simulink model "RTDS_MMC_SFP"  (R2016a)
settings: Solver=FixedStepAuto  StartTime=0.0  StopTime=0.4  RelTol=1e-3
PreLoadFcn:
  | % --- DO NOT REMOVE THIS CODE (2024.3.b1) ---
  |     % create Simulink variants
  |     if not(exist('variant_simulation', 'var'))
  |         variant_simulation = Simulink.Variant('SIMULINK_MODE==0');
  |     end
  |     if not(exist('variant_generation', 'var'))
  |         variant_generation = Simulink.Variant('SIMULINK_MODE==1');
  |     end
  | 
  |     % check SDK version
  |     required_lib_version = 3900.3;
  |     required_lib_ver_str = '2024.3';
  |     lib_path = [getenv('IX_SIMULINK_ACG_BB_3') '\simulink\blocks\BoomBox.slx'];
  |     if exist(lib_path, 'file')
  |         lib_version = str2double(Simulink.MDLInfo(lib_path).ModelVersion); % fullpath to avoid getting shadowing files
  |         if lib_version < required_lib_version || isnan(lib_version)
  |             error(['The model ''' bdroot ''' has been saved with a more recent version of ACG SDK (' required_lib_ver_str ') and might not work as expected. <a href="matlab:private_end_string = ''--- PLACE YOUR CODE BELOW THIS LINE ---'';private_fcn = get_param(bdroot, ''PreLoadFcn'');private_end_index = strfind(private_fcn, private_end_string);set_param(bdroot, ''PreLoadFcn'', strtrim(private_fcn(private_end_index(end)+length(private_end_string):end)));private_fcn = get_param(bdroot, ''PostLoadFcn'');private_end_index = strfind(private_fcn, private_end_string);set_param(bdroot, ''PostLoadFcn'', strtrim(private_fcn(private_end_index(end)+length(private_end_string):end)));private_fcn = get_param(bdroot, ''InitFcn'');private_end_index = strfind(private_fcn, private_end_string);set_param(bdroot, ''InitFcn'', strtrim(private_fcn(private_end_index(end)+length(private_end_string):end)));clear private_end_string private_fcn private_end_index;open(bdroot);">Click here</a> to continue anyway, or download the latest version of the SDK at <a href="www.imperix.com/downloads">www.imperix.ch/downloads</a>.']);
  |         end
  |     elseif exist(getenv('IX_SIMULINK_ACG_BB_3'), 'dir')
  |         error(['Library file for imperix ACG SDK not found in path ''' lib_path '''. Please try to re-install ACG SDK (<a href="www.imperix.com/downloads">www.imperix.ch/downloads</a>).']);
  |     else
  |         error('ACG SDK is not installed on this computer and the model will not work as expected. Please download ACG SDK at <a href="www.imperix.com/downloads">www.imperix.ch/downloads</a>, install it, and reopen the model.');
  |     end
  |     clear required_lib_version required_lib_ver_str lib_path lib_version;
  | 
  |     ix_acg_path = getenv('IX_SIMULINK_ACG_BB_3');
  |     addpath(fullfile(ix_acg_path, 'simulink\target'));
  |     addpath(fullfile(ix_acg_path, 'simulink\blocks'));
  |     addpath(fullfile(ix_acg_path, 'simulink\functions'));
  |     sl_refresh_customizations;
  |     clear ix_acg_path;
  | 
  |     % The SIMULINK_MODE variable is created in the base
  |     % workspace in the PostLoadFcn from the block whose id is kb0101
  |     % All opened models share a common variant configuration.
  | 
  |     Model_PreLoadFcn(bdroot);
  | % --- PLACE YOUR CODE BELOW THIS LINE ---
PostLoadFcn:
  | % --- DO NOT REMOVE THIS CODE (2024.3.b1) ---
  |     % change the execution mode of simulink depending on the radio button:
  |     if(strcmp('Automated Code Generation',get_param(Find_imperix_blocks(bdroot,'Configuration'),'SLMODE')))
  |         assignin('base', 'SIMULINK_MODE', 1);
  |     else
  |         assignin('base', 'SIMULINK_MODE', 0);
  |     end
  | 
  |     Model_PostLoadFcn(bdroot);
  | % --- PLACE YOUR CODE BELOW THIS LINE ---
InitFcn:
  | % --- DO NOT REMOVE THIS CODE (2024.3.b1) ---
  |     % check SDK version
  |     required_lib_version = 3900.3;
  |     required_lib_ver_str = '2024.3';
  |     lib_path = [getenv('IX_SIMULINK_ACG_BB_3') '\simulink\blocks\BoomBox.slx'];
  |     if exist(lib_path, 'file')
  |         lib_version = str2double(Simulink.MDLInfo(lib_path).ModelVersion); % fullpath to avoid getting shadowing files
  |         if lib_version < required_lib_version || isnan(lib_version)
  |             error(['The model ''' bdroot ''' has been saved with a more recent version of ACG SDK (' required_lib_ver_str ') and might not work as expected. <a href="matlab:private_end_string = ''--- PLACE YOUR CODE BELOW THIS LINE ---'';private_fcn = get_param(bdroot, ''PreLoadFcn'');private_end_index = strfind(private_fcn, private_end_string);set_param(bdroot, ''PreLoadFcn'', strtrim(private_fcn(private_end_index(end)+length(private_end_string):end)));private_fcn = get_param(bdroot, ''PostLoadFcn'');private_end_index = strfind(private_fcn, private_end_string);set_param(bdroot, ''PostLoadFcn'', strtrim(private_fcn(private_end_index(end)+length(private_end_string):end)));private_fcn = get_param(bdroot, ''InitFcn'');private_end_index = strfind(private_fcn, private_end_string);set_param(bdroot, ''InitFcn'', strtrim(private_fcn(private_end_index(end)+length(private_end_string):end)));clear private_end_string private_fcn private_end_index;open(bdroot);">Click here</a> to continue anyway, or download the latest version of the SDK at <a href="www.imperix.com/downloads">www.imperix.ch/downloads</a>.']);
  |         end
  |     elseif exist(getenv('IX_SIMULINK_ACG_BB_3'), 'dir')
  |         error(['Library file for imperix ACG SDK not found in path ''' lib_path '''. Please try to re-install ACG SDK (<a href="www.imperix.com/downloads">www.imperix.ch/downloads</a>).']);
  |     else
  |         error('ACG SDK is not installed on this computer and the model will not work as expected. Please download ACG SDK at <a href="www.imperix.com/downloads">www.imperix.ch/downloads</a>, install it, and reopen the model.');
  |     end
  |     clear required_lib_version required_lib_ver_str lib_path lib_version;
  | 
  |     Model_InitFcn(bdroot);
  | % --- PLACE YOUR CODE BELOW THIS LINE ---
model workspace (MAT data in the model file):
  CTRLPERIOD = 0.0002
  TSAMPLE = 2e-06
  global_CLK_number = 0
  global_INT_number = 1
  global_SVM_instance_id = 0
  global_can_baud_rate = '1000000'
  global_comp_time = 0.2
  global_cycle_delay = 8e-05
  global_ip_addresses : cell (value not decoded)
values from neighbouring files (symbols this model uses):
  Ki_Vleg = 1/Ti    (= 2.95256991686)    [RTDS_MMC_SFP_init.m]
  Kp_Vleg = Tn/Ti    (= 0.14880952381)    [RTDS_MMC_SFP_init.m]
  N = 4    [RTDS_MMC_SFP_init.m]
  scale_factor = 0.5^16    (= 1.52587890625e-05)    [RTDS_MMC_SFP_init.m]
  Tsw = 1/fsw    (= 0.0008)    [RTDS_MMC_SFP_init.m]
  Vsm_max = 250    [RTDS_MMC_SFP_init.m]
undefined symbols (not defined in the file or in its folder): B, Board, Box, channel, DT, lane, Micro, ns, PRO, RCP, TPI, Vf
libraries: BoomBox x183, simulink x55
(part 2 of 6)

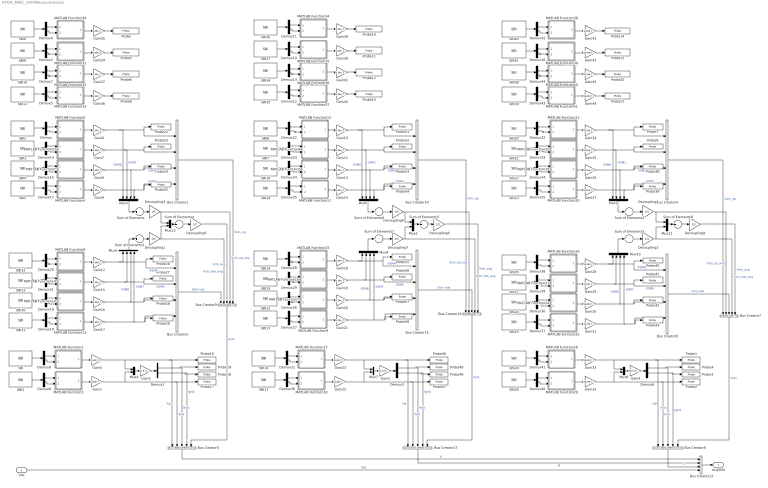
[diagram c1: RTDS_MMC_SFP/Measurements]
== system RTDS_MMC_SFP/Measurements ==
  Vdc : Inport
  Bus Creator{1..2,4,6,13..15} (7 alike) : BusCreator  Inputs=4
  Bus Creator{5,7..9,16..17} (6 alike) : BusCreator  Inputs=5
  Decoupling{1..4,7..8} (6 alike) : Gain  Gain=1/4
  Decoupling5 : Gain  Gain=1/2
  Decoupling6 : Gain  Gain=1/2
  Decoupling9 : Gain  Gain=1/2
  Demux{,1..44} (45 alike) : Demux  Outputs=2
  Gain{1,5..45} (42 alike) : Gain  Gain=scale_factor  OutDataTypeStr=single
  Gain2 : Gain  Gain=[0.5 0.5 ; 1 -1]  Multiplication=Matrix(K*u)
  Gain3 : Gain  Gain=[0.5 0.5 ; 1 -1]  Multiplication=Matrix(K*u)
  Gain4 : Gain  Gain=[0.5 0.5 ; 1 -1]  Multiplication=Matrix(K*u)
  MATLAB Function0 : MATLAB Function  TreatAsAtomicUnit=on
  MATLAB Function1 : MATLAB Function  TreatAsAtomicUnit=on
  MATLAB Function10 : MATLAB Function  TreatAsAtomicUnit=on
  MATLAB Function11 : MATLAB Function  TreatAsAtomicUnit=on
  MATLAB Function12 : MATLAB Function  TreatAsAtomicUnit=on
  MATLAB Function13 : MATLAB Function  TreatAsAtomicUnit=on
  MATLAB Function14 : MATLAB Function  TreatAsAtomicUnit=on
  MATLAB Function15 : MATLAB Function  TreatAsAtomicUnit=on
  MATLAB Function16 : MATLAB Function  TreatAsAtomicUnit=on
  MATLAB Function17 : MATLAB Function  TreatAsAtomicUnit=on
  MATLAB Function18 : MATLAB Function  TreatAsAtomicUnit=on
  MATLAB Function19 : MATLAB Function  TreatAsAtomicUnit=on
  MATLAB Function2 : MATLAB Function  TreatAsAtomicUnit=on
  MATLAB Function20 : MATLAB Function  TreatAsAtomicUnit=on
  MATLAB Function21 : MATLAB Function  TreatAsAtomicUnit=on
  MATLAB Function22 : MATLAB Function  TreatAsAtomicUnit=on
  MATLAB Function23 : MATLAB Function  TreatAsAtomicUnit=on
  MATLAB Function24 : MATLAB Function  TreatAsAtomicUnit=on
  MATLAB Function25 : MATLAB Function  TreatAsAtomicUnit=on
  MATLAB Function26 : MATLAB Function  TreatAsAtomicUnit=on
  MATLAB Function27 : MATLAB Function  TreatAsAtomicUnit=on
  MATLAB Function28 : MATLAB Function  TreatAsAtomicUnit=on
  MATLAB Function29 : MATLAB Function  TreatAsAtomicUnit=on
  MATLAB Function3 : MATLAB Function  TreatAsAtomicUnit=on
  MATLAB Function30 : MATLAB Function  TreatAsAtomicUnit=on
  MATLAB Function31 : MATLAB Function  TreatAsAtomicUnit=on
  MATLAB Function32 : MATLAB Function  TreatAsAtomicUnit=on
  MATLAB Function33 : MATLAB Function  TreatAsAtomicUnit=on
  MATLAB Function34 : MATLAB Function  TreatAsAtomicUnit=on
  MATLAB Function35 : MATLAB Function  TreatAsAtomicUnit=on
  MATLAB Function36 : MATLAB Function  TreatAsAtomicUnit=on
  MATLAB Function37 : MATLAB Function  TreatAsAtomicUnit=on
  MATLAB Function38 : MATLAB Function  TreatAsAtomicUnit=on
  MATLAB Function39 : MATLAB Function  TreatAsAtomicUnit=on
  MATLAB Function4 : MATLAB Function  TreatAsAtomicUnit=on
  MATLAB Function40 : MATLAB Function  TreatAsAtomicUnit=on
  MATLAB Function41 : MATLAB Function  TreatAsAtomicUnit=on
  MATLAB Function5 : MATLAB Function  TreatAsAtomicUnit=on
  MATLAB Function6 : MATLAB Function  TreatAsAtomicUnit=on
  MATLAB Function7 : MATLAB Function  TreatAsAtomicUnit=on
  MATLAB Function8 : MATLAB Function  TreatAsAtomicUnit=on
  MATLAB Function9 : MATLAB Function  TreatAsAtomicUnit=on
  Mux{1,3,5..6,9..10} (6 alike) : Mux
  Mux{2,4,7..8,11..12} (6 alike) : Mux  Inputs=2
  Probe : BoomBox/Probe  VARNAME=v_leg_1  EVALUATE=Literal  DATATYPE=single  CAN_ENABLED=off  CAN_ADDRESS=0  CAN_TX_FREQ=10  init_baudrate=0  CAN_BAUDRATE=1000000  can_endianness=Little-endian  ETH_ENABLED=off  ETH_PORT=2000  ETH_IP_LIST=IP address 0  eth_endianness=Little-endian  ETH_TX_FREQ=10  init_ip=0  KBID=kb0502  CAN_BIG_ENDIAN=0  ETH_BIG_ENDIAN=0  ETH_IP_SFCN=empty  CAN_MB_ID=0  ETH_MB_ID=1  RESIZE=0
  Probe1 : BoomBox/Probe  VARNAME=Iup_C  EVALUATE=Literal  DATATYPE=single  CAN_ENABLED=off  CAN_ADDRESS=0  CAN_TX_FREQ=10  init_baudrate=0  CAN_BAUDRATE=1000000  can_endianness=Little-endian  ETH_ENABLED=off  ETH_PORT=2000  ETH_IP_LIST=IP address 0  eth_endianness=Little-endian  ETH_TX_FREQ=10  init_ip=0  KBID=kb0502  CAN_BIG_ENDIAN=0  ETH_BIG_ENDIAN=0  ETH_IP_SFCN=empty  CAN_MB_ID=0  ETH_MB_ID=0  RESIZE=0
  Probe10 : BoomBox/Probe  VARNAME=v_leg_3  EVALUATE=Literal  DATATYPE=single  CAN_ENABLED=off  CAN_ADDRESS=0  CAN_TX_FREQ=10  init_baudrate=0  CAN_BAUDRATE=1000000  can_endianness=Little-endian  ETH_ENABLED=off  ETH_PORT=2000  ETH_IP_LIST=IP address 0  eth_endianness=Little-endian  ETH_TX_FREQ=10  init_ip=0  KBID=kb0502  CAN_BIG_ENDIAN=0  ETH_BIG_ENDIAN=0  ETH_IP_SFCN=empty  CAN_MB_ID=0  ETH_MB_ID=1  RESIZE=0
  Probe11 : BoomBox/Probe  VARNAME=v_valves_3  EVALUATE=Literal  DATATYPE=single  CAN_ENABLED=off  CAN_ADDRESS=0  CAN_TX_FREQ=10  init_baudrate=0  CAN_BAUDRATE=1000000  can_endianness=Little-endian  ETH_ENABLED=off  ETH_PORT=2000  ETH_IP_LIST=IP address 0  eth_endianness=Little-endian  ETH_TX_FREQ=10  init_ip=0  KBID=kb0502  CAN_BIG_ENDIAN=0  ETH_BIG_ENDIAN=0  ETH_IP_SFCN=empty  CAN_MB_ID=0  ETH_MB_ID=1  RESIZE=0
  Probe12 : BoomBox/Probe  VARNAME=v_leg_4  EVALUATE=Literal  DATATYPE=single  CAN_ENABLED=off  CAN_ADDRESS=0  CAN_TX_FREQ=10  init_baudrate=0  CAN_BAUDRATE=1000000  can_endianness=Little-endian  ETH_ENABLED=off  ETH_PORT=2000  ETH_IP_LIST=IP address 0  eth_endianness=Little-endian  ETH_TX_FREQ=10  init_ip=0  KBID=kb0502  CAN_BIG_ENDIAN=0  ETH_BIG_ENDIAN=0  ETH_IP_SFCN=empty  CAN_MB_ID=0  ETH_MB_ID=1  RESIZE=0
  Probe13 : BoomBox/Probe  VARNAME=v_valves_4  EVALUATE=Literal  DATATYPE=single  CAN_ENABLED=off  CAN_ADDRESS=0  CAN_TX_FREQ=10  init_baudrate=0  CAN_BAUDRATE=1000000  can_endianness=Little-endian  ETH_ENABLED=off  ETH_PORT=2000  ETH_IP_LIST=IP address 0  eth_endianness=Little-endian  ETH_TX_FREQ=10  init_ip=0  KBID=kb0502  CAN_BIG_ENDIAN=0  ETH_BIG_ENDIAN=0  ETH_IP_SFCN=empty  CAN_MB_ID=0  ETH_MB_ID=1  RESIZE=0
  Probe14 : BoomBox/Probe  VARNAME=v_leg_5  EVALUATE=Literal  DATATYPE=single  CAN_ENABLED=off  CAN_ADDRESS=0  CAN_TX_FREQ=10  init_baudrate=0  CAN_BAUDRATE=1000000  can_endianness=Little-endian  ETH_ENABLED=off  ETH_PORT=2000  ETH_IP_LIST=IP address 0  eth_endianness=Little-endian  ETH_TX_FREQ=10  init_ip=0  KBID=kb0502  CAN_BIG_ENDIAN=0  ETH_BIG_ENDIAN=0  ETH_IP_SFCN=empty  CAN_MB_ID=0  ETH_MB_ID=1  RESIZE=0
  Probe15 : BoomBox/Probe  VARNAME=v_valves_5  EVALUATE=Literal  DATATYPE=single  CAN_ENABLED=off  CAN_ADDRESS=0  CAN_TX_FREQ=10  init_baudrate=0  CAN_BAUDRATE=1000000  can_endianness=Little-endian  ETH_ENABLED=off  ETH_PORT=2000  ETH_IP_LIST=IP address 0  eth_endianness=Little-endian  ETH_TX_FREQ=10  init_ip=0  KBID=kb0502  CAN_BIG_ENDIAN=0  ETH_BIG_ENDIAN=0  ETH_IP_SFCN=empty  CAN_MB_ID=0  ETH_MB_ID=1  RESIZE=0
  Probe16 : BoomBox/Probe  VARNAME=Iup_A  EVALUATE=Literal  DATATYPE=single  CAN_ENABLED=off  CAN_ADDRESS=0  CAN_TX_FREQ=10  init_baudrate=0  CAN_BAUDRATE=1000000  can_endianness=Little-endian  ETH_ENABLED=off  ETH_PORT=2000  ETH_IP_LIST=IP address 0  eth_endianness=Little-endian  ETH_TX_FREQ=10  init_ip=0  KBID=kb0502  CAN_BIG_ENDIAN=0  ETH_BIG_ENDIAN=0  ETH_IP_SFCN=empty  CAN_MB_ID=0  ETH_MB_ID=0  RESIZE=0
  Probe17 : BoomBox/Probe  VARNAME=Ilow_A  EVALUATE=Literal  DATATYPE=single  CAN_ENABLED=off  CAN_ADDRESS=0  CAN_TX_FREQ=10  init_baudrate=0  CAN_BAUDRATE=1000000  can_endianness=Little-endian  ETH_ENABLED=off  ETH_PORT=2000  ETH_IP_LIST=IP address 0  eth_endianness=Little-endian  ETH_TX_FREQ=10  init_ip=0  KBID=kb0502  CAN_BIG_ENDIAN=0  ETH_BIG_ENDIAN=0  ETH_IP_SFCN=empty  CAN_MB_ID=0  ETH_MB_ID=0  RESIZE=0
  Probe18 : BoomBox/Probe  VARNAME=Ig_A  EVALUATE=Literal  DATATYPE=single  CAN_ENABLED=off  CAN_ADDRESS=0  CAN_TX_FREQ=10  init_baudrate=0  CAN_BAUDRATE=1000000  can_endianness=Little-endian  ETH_ENABLED=off  ETH_PORT=2000  ETH_IP_LIST=IP address 0  eth_endianness=Little-endian  ETH_TX_FREQ=10  init_ip=0  KBID=kb0502  CAN_BIG_ENDIAN=0  ETH_BIG_ENDIAN=0  ETH_IP_SFCN=empty  CAN_MB_ID=0  ETH_MB_ID=0  RESIZE=0
  Probe19 : BoomBox/Probe  VARNAME=Ibus_A  EVALUATE=Literal  DATATYPE=single  CAN_ENABLED=off  CAN_ADDRESS=0  CAN_TX_FREQ=10  init_baudrate=0  CAN_BAUDRATE=1000000  can_endianness=Little-endian  ETH_ENABLED=off  ETH_PORT=2000  ETH_IP_LIST=IP address 0  eth_endianness=Little-endian  ETH_TX_FREQ=10  init_ip=0  KBID=kb0502  CAN_BIG_ENDIAN=0  ETH_BIG_ENDIAN=0  ETH_IP_SFCN=empty  CAN_MB_ID=0  ETH_MB_ID=0  RESIZE=0
  Probe2 : BoomBox/Probe  VARNAME=Ilow_C  EVALUATE=Literal  DATATYPE=single  CAN_ENABLED=off  CAN_ADDRESS=0  CAN_TX_FREQ=10  init_baudrate=0  CAN_BAUDRATE=1000000  can_endianness=Little-endian  ETH_ENABLED=off  ETH_PORT=2000  ETH_IP_LIST=IP address 0  eth_endianness=Little-endian  ETH_TX_FREQ=10  init_ip=0  KBID=kb0502  CAN_BIG_ENDIAN=0  ETH_BIG_ENDIAN=0  ETH_IP_SFCN=empty  CAN_MB_ID=0  ETH_MB_ID=0  RESIZE=0
  Probe20 : BoomBox/Probe  VARNAME=v_leg_6  EVALUATE=Literal  DATATYPE=single  CAN_ENABLED=off  CAN_ADDRESS=0  CAN_TX_FREQ=10  init_baudrate=0  CAN_BAUDRATE=1000000  can_endianness=Little-endian  ETH_ENABLED=off  ETH_PORT=2000  ETH_IP_LIST=IP address 0  eth_endianness=Little-endian  ETH_TX_FREQ=10  init_ip=0  KBID=kb0502  CAN_BIG_ENDIAN=0  ETH_BIG_ENDIAN=0  ETH_IP_SFCN=empty  CAN_MB_ID=0  ETH_MB_ID=1  RESIZE=0
  Probe21 : BoomBox/Probe  VARNAME=v_valves_6  EVALUATE=Literal  DATATYPE=single  CAN_ENABLED=off  CAN_ADDRESS=0  CAN_TX_FREQ=10  init_baudrate=0  CAN_BAUDRATE=1000000  can_endianness=Little-endian  ETH_ENABLED=off  ETH_PORT=2000  ETH_IP_LIST=IP address 0  eth_endianness=Little-endian  ETH_TX_FREQ=10  init_ip=0  KBID=kb0502  CAN_BIG_ENDIAN=0  ETH_BIG_ENDIAN=0  ETH_IP_SFCN=empty  CAN_MB_ID=0  ETH_MB_ID=1  RESIZE=0
  Probe22 : BoomBox/Probe  VARNAME=Vsm_A0  EVALUATE=Literal  DATATYPE=single  CAN_ENABLED=off  CAN_ADDRESS=0  CAN_TX_FREQ=10  init_baudrate=0  CAN_BAUDRATE=1000000  can_endianness=Little-endian  ETH_ENABLED=off  ETH_PORT=2000  ETH_IP_LIST=IP address 0  eth_endianness=Little-endian  ETH_TX_FREQ=10  init_ip=0  KBID=kb0502  CAN_BIG_ENDIAN=0  ETH_BIG_ENDIAN=0  ETH_IP_SFCN=empty  CAN_MB_ID=0  ETH_MB_ID=0  RESIZE=0
  Probe23 : BoomBox/Probe  VARNAME=Vsm_A1  EVALUATE=Literal  DATATYPE=single  CAN_ENABLED=off  CAN_ADDRESS=0  CAN_TX_FREQ=10  init_baudrate=0  CAN_BAUDRATE=1000000  can_endianness=Little-endian  ETH_ENABLED=off  ETH_PORT=2000  ETH_IP_LIST=IP address 0  eth_endianness=Little-endian  ETH_TX_FREQ=10  init_ip=0  KBID=kb0502  CAN_BIG_ENDIAN=0  ETH_BIG_ENDIAN=0  ETH_IP_SFCN=empty  CAN_MB_ID=0  ETH_MB_ID=0  RESIZE=0
  Probe24 : BoomBox/Probe  VARNAME=Vsm_A2  EVALUATE=Literal  DATATYPE=single  CAN_ENABLED=off  CAN_ADDRESS=0  CAN_TX_FREQ=10  init_baudrate=0  CAN_BAUDRATE=1000000  can_endianness=Little-endian  ETH_ENABLED=off  ETH_PORT=2000  ETH_IP_LIST=IP address 0  eth_endianness=Little-endian  ETH_TX_FREQ=10  init_ip=0  KBID=kb0502  CAN_BIG_ENDIAN=0  ETH_BIG_ENDIAN=0  ETH_IP_SFCN=empty  CAN_MB_ID=0  ETH_MB_ID=0  RESIZE=0
  Probe25 : BoomBox/Probe  VARNAME=Vsm_A3  EVALUATE=Literal  DATATYPE=single  CAN_ENABLED=off  CAN_ADDRESS=0  CAN_TX_FREQ=10  init_baudrate=0  CAN_BAUDRATE=1000000  can_endianness=Little-endian  ETH_ENABLED=off  ETH_PORT=2000  ETH_IP_LIST=IP address 0  eth_endianness=Little-endian  ETH_TX_FREQ=10  init_ip=0  KBID=kb0502  CAN_BIG_ENDIAN=0  ETH_BIG_ENDIAN=0  ETH_IP_SFCN=empty  CAN_MB_ID=0  ETH_MB_ID=0  RESIZE=0
  Probe26 : BoomBox/Probe  VARNAME=Vsm_A4  EVALUATE=Literal  DATATYPE=single  CAN_ENABLED=off  CAN_ADDRESS=0  CAN_TX_FREQ=10  init_baudrate=0  CAN_BAUDRATE=1000000  can_endianness=Little-endian  ETH_ENABLED=off  ETH_PORT=2000  ETH_IP_LIST=IP address 0  eth_endianness=Little-endian  ETH_TX_FREQ=10  init_ip=0  KBID=kb0502  CAN_BIG_ENDIAN=0  ETH_BIG_ENDIAN=0  ETH_IP_SFCN=empty  CAN_MB_ID=0  ETH_MB_ID=0  RESIZE=0
  Probe27 : BoomBox/Probe  VARNAME=Vsm_A5  EVALUATE=Literal  DATATYPE=single  CAN_ENABLED=off  CAN_ADDRESS=0  CAN_TX_FREQ=10  init_baudrate=0  CAN_BAUDRATE=1000000  can_endianness=Little-endian  ETH_ENABLED=off  ETH_PORT=2000  ETH_IP_LIST=IP address 0  eth_endianness=Little-endian  ETH_TX_FREQ=10  init_ip=0  KBID=kb0502  CAN_BIG_ENDIAN=0  ETH_BIG_ENDIAN=0  ETH_IP_SFCN=empty  CAN_MB_ID=0  ETH_MB_ID=0  RESIZE=0
  Probe28 : BoomBox/Probe  VARNAME=Vsm_A6  EVALUATE=Literal  DATATYPE=single  CAN_ENABLED=off  CAN_ADDRESS=0  CAN_TX_FREQ=10  init_baudrate=0  CAN_BAUDRATE=1000000  can_endianness=Little-endian  ETH_ENABLED=off  ETH_PORT=2000  ETH_IP_LIST=IP address 0  eth_endianness=Little-endian  ETH_TX_FREQ=10  init_ip=0  KBID=kb0502  CAN_BIG_ENDIAN=0  ETH_BIG_ENDIAN=0  ETH_IP_SFCN=empty  CAN_MB_ID=0  ETH_MB_ID=0  RESIZE=0
  Probe29 : BoomBox/Probe  VARNAME=Vsm_A7  EVALUATE=Literal  DATATYPE=single  CAN_ENABLED=off  CAN_ADDRESS=0  CAN_TX_FREQ=10  init_baudrate=0  CAN_BAUDRATE=1000000  can_endianness=Little-endian  ETH_ENABLED=off  ETH_PORT=2000  ETH_IP_LIST=IP address 0  eth_endianness=Little-endian  ETH_TX_FREQ=10  init_ip=0  KBID=kb0502  CAN_BIG_ENDIAN=0  ETH_BIG_ENDIAN=0  ETH_IP_SFCN=empty  CAN_MB_ID=0  ETH_MB_ID=0  RESIZE=0
  Probe3 : BoomBox/Probe  VARNAME=Ig_C  EVALUATE=Literal  DATATYPE=single  CAN_ENABLED=off  CAN_ADDRESS=0  CAN_TX_FREQ=10  init_baudrate=0  CAN_BAUDRATE=1000000  can_endianness=Little-endian  ETH_ENABLED=off  ETH_PORT=2000  ETH_IP_LIST=IP address 0  eth_endianness=Little-endian  ETH_TX_FREQ=10  init_ip=0  KBID=kb0502  CAN_BIG_ENDIAN=0  ETH_BIG_ENDIAN=0  ETH_IP_SFCN=empty  CAN_MB_ID=0  ETH_MB_ID=0  RESIZE=0
  Probe38 : BoomBox/Probe  VARNAME=Vsm_C2  EVALUATE=Literal  DATATYPE=single  CAN_ENABLED=off  CAN_ADDRESS=0  CAN_TX_FREQ=10  init_baudrate=0  CAN_BAUDRATE=1000000  can_endianness=Little-endian  ETH_ENABLED=off  ETH_PORT=2000  ETH_IP_LIST=IP address 0  eth_endianness=Little-endian  ETH_TX_FREQ=10  init_ip=0  KBID=kb0502  CAN_BIG_ENDIAN=0  ETH_BIG_ENDIAN=0  ETH_IP_SFCN=empty  CAN_MB_ID=0  ETH_MB_ID=0  RESIZE=0
  Probe39 : BoomBox/Probe  VARNAME=Vsm_C3  EVALUATE=Literal  DATATYPE=single  CAN_ENABLED=off  CAN_ADDRESS=0  CAN_TX_FREQ=10  init_baudrate=0  CAN_BAUDRATE=1000000  can_endianness=Little-endian  ETH_ENABLED=off  ETH_PORT=2000  ETH_IP_LIST=IP address 0  eth_endianness=Little-endian  ETH_TX_FREQ=10  init_ip=0  KBID=kb0502  CAN_BIG_ENDIAN=0  ETH_BIG_ENDIAN=0  ETH_IP_SFCN=empty  CAN_MB_ID=0  ETH_MB_ID=0  RESIZE=0
  Probe4 : BoomBox/Probe  VARNAME=Ibus_C  EVALUATE=Literal  DATATYPE=single  CAN_ENABLED=off  CAN_ADDRESS=0  CAN_TX_FREQ=10  init_baudrate=0  CAN_BAUDRATE=1000000  can_endianness=Little-endian  ETH_ENABLED=off  ETH_PORT=2000  ETH_IP_LIST=IP address 0  eth_endianness=Little-endian  ETH_TX_FREQ=10  init_ip=0  KBID=kb0502  CAN_BIG_ENDIAN=0  ETH_BIG_ENDIAN=0  ETH_IP_SFCN=empty  CAN_MB_ID=0  ETH_MB_ID=0  RESIZE=0
  Probe40 : BoomBox/Probe  VARNAME=Vsm_C4  EVALUATE=Literal  DATATYPE=single  CAN_ENABLED=off  CAN_ADDRESS=0  CAN_TX_FREQ=10  init_baudrate=0  CAN_BAUDRATE=1000000  can_endianness=Little-endian  ETH_ENABLED=off  ETH_PORT=2000  ETH_IP_LIST=IP address 0  eth_endianness=Little-endian  ETH_TX_FREQ=10  init_ip=0  KBID=kb0502  CAN_BIG_ENDIAN=0  ETH_BIG_ENDIAN=0  ETH_IP_SFCN=empty  CAN_MB_ID=0  ETH_MB_ID=0  RESIZE=0
  Probe41 : BoomBox/Probe  VARNAME=Vsm_C5  EVALUATE=Literal  DATATYPE=single  CAN_ENABLED=off  CAN_ADDRESS=0  CAN_TX_FREQ=10  init_baudrate=0  CAN_BAUDRATE=1000000  can_endianness=Little-endian  ETH_ENABLED=off  ETH_PORT=2000  ETH_IP_LIST=IP address 0  eth_endianness=Little-endian  ETH_TX_FREQ=10  init_ip=0  KBID=kb0502  CAN_BIG_ENDIAN=0  ETH_BIG_ENDIAN=0  ETH_IP_SFCN=empty  CAN_MB_ID=0  ETH_MB_ID=0  RESIZE=0
  Probe42 : BoomBox/Probe  VARNAME=Vsm_C6  EVALUATE=Literal  DATATYPE=single  CAN_ENABLED=off  CAN_ADDRESS=0  CAN_TX_FREQ=10  init_baudrate=0  CAN_BAUDRATE=1000000  can_endianness=Little-endian  ETH_ENABLED=off  ETH_PORT=2000  ETH_IP_LIST=IP address 0  eth_endianness=Little-endian  ETH_TX_FREQ=10  init_ip=0  KBID=kb0502  CAN_BIG_ENDIAN=0  ETH_BIG_ENDIAN=0  ETH_IP_SFCN=empty  CAN_MB_ID=0  ETH_MB_ID=0  RESIZE=0
  Probe43 : BoomBox/Probe  VARNAME=Vsm_C7  EVALUATE=Literal  DATATYPE=single  CAN_ENABLED=off  CAN_ADDRESS=0  CAN_TX_FREQ=10  init_baudrate=0  CAN_BAUDRATE=1000000  can_endianness=Little-endian  ETH_ENABLED=off  ETH_PORT=2000  ETH_IP_LIST=IP address 0  eth_endianness=Little-endian  ETH_TX_FREQ=10  init_ip=0  KBID=kb0502  CAN_BIG_ENDIAN=0  ETH_BIG_ENDIAN=0  ETH_IP_SFCN=empty  CAN_MB_ID=0  ETH_MB_ID=0  RESIZE=0
  Probe46 : BoomBox/Probe  VARNAME=Iup_B  EVALUATE=Literal  DATATYPE=single  CAN_ENABLED=off  CAN_ADDRESS=0  CAN_TX_FREQ=10  init_baudrate=0  CAN_BAUDRATE=1000000  can_endianness=Little-endian  ETH_ENABLED=off  ETH_PORT=2000  ETH_IP_LIST=IP address 0  eth_endianness=Little-endian  ETH_TX_FREQ=10  init_ip=0  KBID=kb0502  CAN_BIG_ENDIAN=0  ETH_BIG_ENDIAN=0  ETH_IP_SFCN=empty  CAN_MB_ID=0  ETH_MB_ID=0  RESIZE=0
  Probe47 : BoomBox/Probe  VARNAME=Ilow_B  EVALUATE=Literal  DATATYPE=single  CAN_ENABLED=off  CAN_ADDRESS=0  CAN_TX_FREQ=10  init_baudrate=0  CAN_BAUDRATE=1000000  can_endianness=Little-endian  ETH_ENABLED=off  ETH_PORT=2000  ETH_IP_LIST=IP address 0  eth_endianness=Little-endian  ETH_TX_FREQ=10  init_ip=0  KBID=kb0502  CAN_BIG_ENDIAN=0  ETH_BIG_ENDIAN=0  ETH_IP_SFCN=empty  CAN_MB_ID=0  ETH_MB_ID=0  RESIZE=0
  Probe48 : BoomBox/Probe  VARNAME=Ig_B  EVALUATE=Literal  DATATYPE=single  CAN_ENABLED=off  CAN_ADDRESS=0  CAN_TX_FREQ=10  init_baudrate=0  CAN_BAUDRATE=1000000  can_endianness=Little-endian  ETH_ENABLED=off  ETH_PORT=2000  ETH_IP_LIST=IP address 0  eth_endianness=Little-endian  ETH_TX_FREQ=10  init_ip=0  KBID=kb0502  CAN_BIG_ENDIAN=0  ETH_BIG_ENDIAN=0  ETH_IP_SFCN=empty  CAN_MB_ID=0  ETH_MB_ID=0  RESIZE=0
  Probe49 : BoomBox/Probe  VARNAME=Ibus_B  EVALUATE=Literal  DATATYPE=single  CAN_ENABLED=off  CAN_ADDRESS=0  CAN_TX_FREQ=10  init_baudrate=0  CAN_BAUDRATE=1000000  can_endianness=Little-endian  ETH_ENABLED=off  ETH_PORT=2000  ETH_IP_LIST=IP address 0  eth_endianness=Little-endian  ETH_TX_FREQ=10  init_ip=0  KBID=kb0502  CAN_BIG_ENDIAN=0  ETH_BIG_ENDIAN=0  ETH_IP_SFCN=empty  CAN_MB_ID=0  ETH_MB_ID=0  RESIZE=0
  Probe5 : BoomBox/Probe  VARNAME=v_valves_1  EVALUATE=Literal  DATATYPE=single  CAN_ENABLED=off  CAN_ADDRESS=0  CAN_TX_FREQ=10  init_baudrate=0  CAN_BAUDRATE=1000000  can_endianness=Little-endian  ETH_ENABLED=off  ETH_PORT=2000  ETH_IP_LIST=IP address 0  eth_endianness=Little-endian  ETH_TX_FREQ=10  init_ip=0  KBID=kb0502  CAN_BIG_ENDIAN=0  ETH_BIG_ENDIAN=0  ETH_IP_SFCN=empty  CAN_MB_ID=0  ETH_MB_ID=1  RESIZE=0
  Probe51 : BoomBox/Probe  VARNAME=Vsm_B0  EVALUATE=Literal  DATATYPE=single  CAN_ENABLED=off  CAN_ADDRESS=0  CAN_TX_FREQ=10  init_baudrate=0  CAN_BAUDRATE=1000000  can_endianness=Little-endian  ETH_ENABLED=off  ETH_PORT=2000  ETH_IP_LIST=IP address 0  eth_endianness=Little-endian  ETH_TX_FREQ=10  init_ip=0  KBID=kb0502  CAN_BIG_ENDIAN=0  ETH_BIG_ENDIAN=0  ETH_IP_SFCN=empty  CAN_MB_ID=0  ETH_MB_ID=0  RESIZE=0
  Probe52 : BoomBox/Probe  VARNAME=Vsm_B1  EVALUATE=Literal  DATATYPE=single  CAN_ENABLED=off  CAN_ADDRESS=0  CAN_TX_FREQ=10  init_baudrate=0  CAN_BAUDRATE=1000000  can_endianness=Little-endian  ETH_ENABLED=off  ETH_PORT=2000  ETH_IP_LIST=IP address 0  eth_endianness=Little-endian  ETH_TX_FREQ=10  init_ip=0  KBID=kb0502  CAN_BIG_ENDIAN=0  ETH_BIG_ENDIAN=0  ETH_IP_SFCN=empty  CAN_MB_ID=0  ETH_MB_ID=0  RESIZE=0
  Probe53 : BoomBox/Probe  VARNAME=Vsm_B2  EVALUATE=Literal  DATATYPE=single  CAN_ENABLED=off  CAN_ADDRESS=0  CAN_TX_FREQ=10  init_baudrate=0  CAN_BAUDRATE=1000000  can_endianness=Little-endian  ETH_ENABLED=off  ETH_PORT=2000  ETH_IP_LIST=IP address 0  eth_endianness=Little-endian  ETH_TX_FREQ=10  init_ip=0  KBID=kb0502  CAN_BIG_ENDIAN=0  ETH_BIG_ENDIAN=0  ETH_IP_SFCN=empty  CAN_MB_ID=0  ETH_MB_ID=0  RESIZE=0
  Probe54 : BoomBox/Probe  VARNAME=Vsm_B3  EVALUATE=Literal  DATATYPE=single  CAN_ENABLED=off  CAN_ADDRESS=0  CAN_TX_FREQ=10  init_baudrate=0  CAN_BAUDRATE=1000000  can_endianness=Little-endian  ETH_ENABLED=off  ETH_PORT=2000  ETH_IP_LIST=IP address 0  eth_endianness=Little-endian  ETH_TX_FREQ=10  init_ip=0  KBID=kb0502  CAN_BIG_ENDIAN=0  ETH_BIG_ENDIAN=0  ETH_IP_SFCN=empty  CAN_MB_ID=0  ETH_MB_ID=0  RESIZE=0
  Probe55 : BoomBox/Probe  VARNAME=Vsm_B4  EVALUATE=Literal  DATATYPE=single  CAN_ENABLED=off  CAN_ADDRESS=0  CAN_TX_FREQ=10  init_baudrate=0  CAN_BAUDRATE=1000000  can_endianness=Little-endian  ETH_ENABLED=off  ETH_PORT=2000  ETH_IP_LIST=IP address 0  eth_endianness=Little-endian  ETH_TX_FREQ=10  init_ip=0  KBID=kb0502  CAN_BIG_ENDIAN=0  ETH_BIG_ENDIAN=0  ETH_IP_SFCN=empty  CAN_MB_ID=0  ETH_MB_ID=0  RESIZE=0
  Probe56 : BoomBox/Probe  VARNAME=Vsm_B5  EVALUATE=Literal  DATATYPE=single  CAN_ENABLED=off  CAN_ADDRESS=0  CAN_TX_FREQ=10  init_baudrate=0  CAN_BAUDRATE=1000000  can_endianness=Little-endian  ETH_ENABLED=off  ETH_PORT=2000  ETH_IP_LIST=IP address 0  eth_endianness=Little-endian  ETH_TX_FREQ=10  init_ip=0  KBID=kb0502  CAN_BIG_ENDIAN=0  ETH_BIG_ENDIAN=0  ETH_IP_SFCN=empty  CAN_MB_ID=0  ETH_MB_ID=0  RESIZE=0
  Probe57 : BoomBox/Probe  VARNAME=Vsm_B6  EVALUATE=Literal  DATATYPE=single  CAN_ENABLED=off  CAN_ADDRESS=0  CAN_TX_FREQ=10  init_baudrate=0  CAN_BAUDRATE=1000000  can_endianness=Little-endian  ETH_ENABLED=off  ETH_PORT=2000  ETH_IP_LIST=IP address 0  eth_endianness=Little-endian  ETH_TX_FREQ=10  init_ip=0  KBID=kb0502  CAN_BIG_ENDIAN=0  ETH_BIG_ENDIAN=0  ETH_IP_SFCN=empty  CAN_MB_ID=0  ETH_MB_ID=0  RESIZE=0
  Probe58 : BoomBox/Probe  VARNAME=Vsm_B7  EVALUATE=Literal  DATATYPE=single  CAN_ENABLED=off  CAN_ADDRESS=0  CAN_TX_FREQ=10  init_baudrate=0  CAN_BAUDRATE=1000000  can_endianness=Little-endian  ETH_ENABLED=off  ETH_PORT=2000  ETH_IP_LIST=IP address 0  eth_endianness=Little-endian  ETH_TX_FREQ=10  init_ip=0  KBID=kb0502  CAN_BIG_ENDIAN=0  ETH_BIG_ENDIAN=0  ETH_IP_SFCN=empty  CAN_MB_ID=0  ETH_MB_ID=0  RESIZE=0
  Probe6 : BoomBox/Probe  VARNAME=v_leg_2  EVALUATE=Literal  DATATYPE=single  CAN_ENABLED=off  CAN_ADDRESS=0  CAN_TX_FREQ=10  init_baudrate=0  CAN_BAUDRATE=1000000  can_endianness=Little-endian  ETH_ENABLED=off  ETH_PORT=2000  ETH_IP_LIST=IP address 0  eth_endianness=Little-endian  ETH_TX_FREQ=10  init_ip=0  KBID=kb0502  CAN_BIG_ENDIAN=0  ETH_BIG_ENDIAN=0  ETH_IP_SFCN=empty  CAN_MB_ID=0  ETH_MB_ID=1  RESIZE=0
  Probe7 : BoomBox/Probe  VARNAME=Vsm_C0  EVALUATE=Literal  DATATYPE=single  CAN_ENABLED=off  CAN_ADDRESS=0  CAN_TX_FREQ=10  init_baudrate=0  CAN_BAUDRATE=1000000  can_endianness=Little-endian  ETH_ENABLED=off  ETH_PORT=2000  ETH_IP_LIST=IP address 0  eth_endianness=Little-endian  ETH_TX_FREQ=10  init_ip=0  KBID=kb0502  CAN_BIG_ENDIAN=0  ETH_BIG_ENDIAN=0  ETH_IP_SFCN=empty  CAN_MB_ID=0  ETH_MB_ID=0  RESIZE=0
  Probe8 : BoomBox/Probe  VARNAME=v_valves_2  EVALUATE=Literal  DATATYPE=single  CAN_ENABLED=off  CAN_ADDRESS=0  CAN_TX_FREQ=10  init_baudrate=0  CAN_BAUDRATE=1000000  can_endianness=Little-endian  ETH_ENABLED=off  ETH_PORT=2000  ETH_IP_LIST=IP address 0  eth_endianness=Little-endian  ETH_TX_FREQ=10  init_ip=0  KBID=kb0502  CAN_BIG_ENDIAN=0  ETH_BIG_ENDIAN=0  ETH_IP_SFCN=empty  CAN_MB_ID=0  ETH_MB_ID=1  RESIZE=0
  Probe9 : BoomBox/Probe  VARNAME=Vsm_C1  EVALUATE=Literal  DATATYPE=single  CAN_ENABLED=off  CAN_ADDRESS=0  CAN_TX_FREQ=10  init_baudrate=0  CAN_BAUDRATE=1000000  can_endianness=Little-endian  ETH_ENABLED=off  ETH_PORT=2000  ETH_IP_LIST=IP address 0  eth_endianness=Little-endian  ETH_TX_FREQ=10  init_ip=0  KBID=kb0502  CAN_BIG_ENDIAN=0  ETH_BIG_ENDIAN=0  ETH_IP_SFCN=empty  CAN_MB_ID=0  ETH_MB_ID=0  RESIZE=0
  SBI : BoomBox/SBI  NB_BBX=0  START_REG=02  NB_REG=2  SIM_IN=off  KBID=kb0209
  SBI1 : BoomBox/SBI  NB_BBX=0  START_REG=08  NB_REG=2  SIM_IN=off  KBID=kb0209
  SBI10 : BoomBox/SBI  NB_BBX=0  START_REG=06  NB_REG=2  SIM_IN=off  KBID=kb0209
  SBI11 : BoomBox/SBI  NB_BBX=0  START_REG=10  NB_REG=2  SIM_IN=off  KBID=kb0209
  SBI12 : BoomBox/SBI  NB_BBX=0  START_REG=88  NB_REG=2  SIM_IN=off  KBID=kb0209
  SBI13 : BoomBox/SBI  NB_BBX=0  START_REG=90  NB_REG=2  SIM_IN=off  KBID=kb0209
  SBI14 : BoomBox/SBI  NB_BBX=0  START_REG=84  NB_REG=2  SIM_IN=off  KBID=kb0209
  SBI15 : BoomBox/SBI  NB_BBX=0  START_REG=86  NB_REG=2  SIM_IN=off  KBID=kb0209
  SBI16 : BoomBox/SBI  NB_BBX=0  START_REG=14  NB_REG=2  SIM_IN=off  KBID=kb0209
  SBI17 : BoomBox/SBI  NB_BBX=0  START_REG=20  NB_REG=2  SIM_IN=off  KBID=kb0209
  SBI18 : BoomBox/SBI  NB_BBX=0  START_REG=80  NB_REG=2  SIM_IN=off  KBID=kb0209
  SBI19 : BoomBox/SBI  NB_BBX=0  START_REG=82  NB_REG=2  SIM_IN=off  KBID=kb0209
  SBI2 : BoomBox/SBI  NB_BBX=0  START_REG=60  NB_REG=2  SIM_IN=off  KBID=kb0209
  SBI20 : BoomBox/SBI  NB_BBX=0  START_REG=92  NB_REG=2  SIM_IN=off  KBID=kb0209
  SBI21 : BoomBox/SBI  NB_BBX=0  START_REG=94  NB_REG=2  SIM_IN=off  KBID=kb0209
  SBI22 : BoomBox/SBI  NB_BBX=0  START_REG=96  NB_REG=2  SIM_IN=off  KBID=kb0209
  SBI23 : BoomBox/SBI  NB_BBX=0  START_REG=98  NB_REG=2  SIM_IN=off  KBID=kb0209
  SBI24 : BoomBox/SBI  NB_BBX=0  START_REG=104  NB_REG=2  SIM_IN=off  KBID=kb0209
  SBI25 : BoomBox/SBI  NB_BBX=0  START_REG=106  NB_REG=2  SIM_IN=off  KBID=kb0209
  SBI26 : BoomBox/SBI  NB_BBX=0  START_REG=100  NB_REG=2  SIM_IN=off  KBID=kb0209
  SBI27 : BoomBox/SBI  NB_BBX=0  START_REG=102  NB_REG=2  SIM_IN=off  KBID=kb0209
  SBI28 : BoomBox/SBI  NB_BBX=0  START_REG=26  NB_REG=2  SIM_IN=off  KBID=kb0209
  SBI29 : BoomBox/SBI  NB_BBX=0  START_REG=32  NB_REG=2  SIM_IN=off  KBID=kb0209
  SBI3 : BoomBox/SBI  NB_BBX=0  START_REG=62  NB_REG=2  SIM_IN=off  KBID=kb0209
  SBI30 : BoomBox/SBI  NB_BBX=0  START_REG=72  NB_REG=2  SIM_IN=off  KBID=kb0209
  SBI31 : BoomBox/SBI  NB_BBX=0  START_REG=74  NB_REG=2  SIM_IN=off  KBID=kb0209
  SBI32 : BoomBox/SBI  NB_BBX=0  START_REG=68  NB_REG=2  SIM_IN=off  KBID=kb0209
  SBI33 : BoomBox/SBI  NB_BBX=0  START_REG=70  NB_REG=2  SIM_IN=off  KBID=kb0209
  SBI34 : BoomBox/SBI  NB_BBX=0  START_REG=18  NB_REG=2  SIM_IN=off  KBID=kb0209
  SBI35 : BoomBox/SBI  NB_BBX=0  START_REG=22  NB_REG=2  SIM_IN=off  KBID=kb0209
  SBI36 : BoomBox/SBI  NB_BBX=0  START_REG=12  NB_REG=2  SIM_IN=off  KBID=kb0209
  SBI37 : BoomBox/SBI  NB_BBX=0  START_REG=16  NB_REG=2  SIM_IN=off  KBID=kb0209
  SBI38 : BoomBox/SBI  NB_BBX=0  START_REG=30  NB_REG=2  SIM_IN=off  KBID=kb0209
  SBI39 : BoomBox/SBI  NB_BBX=0  START_REG=34  NB_REG=2  SIM_IN=off  KBID=kb0209
  SBI4 : BoomBox/SBI  NB_BBX=0  START_REG=64  NB_REG=2  SIM_IN=off  KBID=kb0209
  SBI40 : BoomBox/SBI  NB_BBX=0  START_REG=24  NB_REG=2  SIM_IN=off  KBID=kb0209
  SBI41 : BoomBox/SBI  NB_BBX=0  START_REG=28  NB_REG=2  SIM_IN=off  KBID=kb0209
  SBI5 : BoomBox/SBI  NB_BBX=0  START_REG=66  NB_REG=2  SIM_IN=off  KBID=kb0209
  SBI6 : BoomBox/SBI  NB_BBX=0  START_REG=76  NB_REG=2  SIM_IN=off  KBID=kb0209
  SBI7 : BoomBox/SBI  NB_BBX=0  START_REG=78  NB_REG=2  SIM_IN=off  KBID=kb0209
  SBI8 : BoomBox/SBI  NB_BBX=0  START_REG=00  NB_REG=2  SIM_IN=off  KBID=kb0209
  SBI9 : BoomBox/SBI  NB_BBX=0  START_REG=04  NB_REG=2  SIM_IN=off  KBID=kb0209
  Sum of Elements{,1..8} (9 alike) : Sum  Inputs=+
  acqdata : Outport
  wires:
  Mux8/1 -> Gain4/1
  Demux1/1 -> Probe19/1, Bus Creator5/3  "Ibus"
  Sum of Elements2/1 -> Decoupling4/1
  Sum of Elements6/1 -> Decoupling8/1
  Gain22/1 -> Mux7/2, Probe47/1, Bus Creator17/2  "Ilow"
  Gain33/1 -> Probe1/1, Bus Creator8/1, Mux8/1  "Iup"
  Gain3/1 -> Demux1/1
  Demux6/2 -> Probe3/1, Bus Creator8/4  "Igrid"
  Mux3/1 -> Sum of Elements/1
  Sum of Elements7/1 -> Decoupling7/1
  Bus Creator7/1 -> Bus Creator8/5  "Vsm"
  Gain23/1 -> Probe46/1, Bus Creator17/1, Mux7/1  "Iup"
  Gain5/1 -> Probe16/1, Bus Creator5/1, Mux4/1  "Iup"
  Gain4/1 -> Demux6/1
  Decoupling8/1 -> Bus Creator16/2, Mux2/1  "Vsm_up_avg"
  Bus Creator4/1 -> Bus Creator7/1  "Vsm_up"
  Bus Creator8/1 -> Bus Creator13/3  "C"
  Bus Creator5/1 -> Bus Creator13/1  "A"
  Bus Creator13/1 -> acqdata/1
  Bus Creator6/1 -> Bus Creator7/3  "Vsm_low"
  Bus Creator15/1 -> Bus Creator16/3  "Vsm_low"
  Mux7/1 -> Gain2/1
  Gain1/1 -> Mux4/2, Probe17/1, Bus Creator5/2  "Ilow"
  Bus Creator17/1 -> Bus Creator13/2  "B"
  Decoupling7/1 -> Bus Creator16/4, Mux2/2  "Vsm_low_avg"
  Vdc/1 -> Bus Creator13/4  "Vdc"
  Mux4/1 -> Gain3/1
  Decoupling2/1 -> Bus Creator7/4, Mux11/2  "Vsm_low_avg"
  Mux1/1 -> Sum of Elements2/1
  Mux9/1 -> Sum of Elements7/1
  Bus Creator16/1 -> Bus Creator17/5  "Vsm"
  Sum of Elements/1 -> Decoupling3/1
  Demux6/1 -> Probe4/1, Bus Creator8/3  "Ibus"
  Sum of Elements1/1 -> Decoupling1/1
  Demux1/2 -> Probe18/1, Bus Creator5/4  "Igrid"
  Demux3/1 -> Probe49/1, Bus Creator17/3  "Ibus"
  Gain2/1 -> Demux3/1
  Mux10/1 -> Sum of Elements3/1
  Mux6/1 -> Sum of Elements6/1
  Bus Creator14/1 -> Bus Creator16/1  "Vsm_up"
  Sum of Elements3/1 -> Decoupling2/1
  Mux5/1 -> Sum of Elements1/1
  Gain32/1 -> Mux8/2, Probe2/1, Bus Creator8/2  "Ilow"
  Demux3/2 -> Probe48/1, Bus Creator17/4  "Igrid"
  Decoupling6/1 -> Bus Creator16/5  "Vsm_avg"
  Mux2/1 -> Sum of Elements5/1
  Mux11/1 -> Sum of Elements8/1
  Decoupling4/1 -> Bus Creator7/2, Mux11/1  "Vsm_up_avg"
  Decoupling9/1 -> Bus Creator7/5  "Vsm_avg"
  Bus Creator9/1 -> Bus Creator5/5  "Vsm"
  Mux12/1 -> Sum of Elements4/1
  Sum of Elements4/1 -> Decoupling5/1
  Bus Creator1/1 -> Bus Creator9/5  "Vsm_up"
  Decoupling3/1 -> Mux12/1, Bus Creator9/4  "Vsm_up_avg"
  Decoupling5/1 -> Bus Creator9/3  "Vsm_avg"
  Decoupling1/1 -> Mux12/2, Bus Creator9/2  "Vsm_low_avg"
  Bus Creator2/1 -> Bus Creator9/1  "Vsm_low"
  Sum of Elements5/1 -> Decoupling6/1
  Sum of Elements8/1 -> Decoupling9/1
  Gain12/1 -> Mux5/1, Probe26/1, Bus Creator2/1  "VSM4"
  Gain15/1 -> Mux5/2, Probe27/1, Bus Creator2/2  "VSM5"
  Gain16/1 -> Mux5/3, Probe28/1, Bus Creator2/3  "VSM6"
  Gain17/1 -> Mux5/4, Bus Creator2/4, Probe29/1  "VSM7"
  Gain6/1 -> Probe22/1, Bus Creator1/1, Mux3/1  "VSM0"
  Gain8/1 -> Probe24/1, Bus Creator1/3, Mux3/3  "VSM2"
  Gain9/1 -> Probe25/1, Bus Creator1/4, Mux3/4  "VSM3"
  Gain7/1 -> Bus Creator1/2, Probe23/1, Mux3/2  "VSM1"
  Gain18/1 -> Bus Creator15/1, Probe55/1, Mux9/1  "VSM4"
  Gain20/1 -> Probe57/1, Bus Creator15/3, Mux9/3  "VSM6"
  Gain19/1 -> Bus Creator15/2, Probe56/1, Mux9/2  "VSM5"
  Gain10/1 -> Probe51/1, Bus Creator14/1, Mux6/1  "VSM0"
  Gain21/1 -> Bus Creator15/4, Probe58/1, Mux9/4  "VSM7"
  Gain11/1 -> Bus Creator14/2, Probe52/1, Mux6/2  "VSM1"
  Gain13/1 -> Probe53/1, Bus Creator14/3, Mux6/3  "VSM2"
  Gain14/1 -> Probe54/1, Bus Creator14/4, Mux6/4  "VSM3"
  Gain31/1 -> Bus Creator6/4, Probe43/1, Mux10/4  "VSM7"
  Gain28/1 -> Probe40/1, Bus Creator6/1, Mux10/1  "VSM4"
  Gain29/1 -> Probe41/1, Bus Creator6/2, Mux10/2  "VSM5"
  Gain30/1 -> Bus Creator6/3, Probe42/1, Mux10/3  "VSM6"
  Gain27/1 -> Probe39/1, Bus Creator4/4, Mux1/4  "VSM3"
  Gain26/1 -> Probe38/1, Bus Creator4/3, Mux1/3  "VSM2"
  Gain25/1 -> Mux1/2, Bus Creator4/2, Probe9/1  "VSM1"
  Gain24/1 -> Probe7/1, Bus Creator4/1, Mux1/1  "VSM0"
  MATLAB Function3/1(y) -> Gain1/1
  Demux8/1 -> MATLAB Function3/1(u1)
  SBI1/1 -> Demux8/1
  Demux8/2 -> MATLAB Function3/2(u2)
  MATLAB Function1/1(y) -> Gain5/1
  SBI/1 -> Demux9/1
  Demux9/1 -> MATLAB Function1/1(u1)
  Demux9/2 -> MATLAB Function1/2(u2)
  MATLAB Function4/1(y) -> Gain9/1
  MATLAB Function0/1(y) -> Gain6/1
  MATLAB Function2/1(y) -> Gain8/1
  MATLAB Function23/1(y) -> Gain7/1
  Demux/1 -> MATLAB Function0/1(u1)
  Demux/2 -> MATLAB Function0/2(u2)
  SBI2/1 -> Demux/1
  SBI3/1 -> Demux14/1
  Demux14/2 -> MATLAB Function23/2(u2)
  Demux14/1 -> MATLAB Function23/1(u1)
  Demux17/1 -> MATLAB Function4/1(u1)
  Demux17/2 -> MATLAB Function4/2(u2)
  SBI5/1 -> Demux17/1
  SBI4/1 -> Demux15/1
  Demux15/2 -> MATLAB Function2/2(u2)
  Demux15/1 -> MATLAB Function2/1(u1)
  MATLAB Function13/1(y) -> Gain17/1
  MATLAB Function8/1(y) -> Gain12/1
  Demux19/1 -> MATLAB Function13/1(u1)
  Demux20/1 -> MATLAB Function8/1(u1)
  SBI30/1 -> Demux18/1
  MATLAB Function10/1(y) -> Gain16/1
  Demux21/2 -> MATLAB Function14/2(u2)
  SBI32/1 -> Demux20/1
  MATLAB Function14/1(y) -> Gain15/1
  SBI31/1 -> Demux19/1
  Demux21/1 -> MATLAB Function14/1(u1)
  Demux18/2 -> MATLAB Function10/2(u2)
  Demux20/2 -> MATLAB Function8/2(u2)
  SBI33/1 -> Demux21/1
  Demux18/1 -> MATLAB Function10/1(u1)
  Demux19/2 -> MATLAB Function13/2(u2)
  MATLAB Function11/1(y) -> Gain14/1
  MATLAB Function12/1(y) -> Gain10/1
  MATLAB Function5/1(y) -> Gain13/1
  MATLAB Function6/1(y) -> Gain11/1
  Demux22/2 -> MATLAB Function12/2(u2)
  SBI6/1 -> Demux22/1
  SBI7/1 -> Demux23/1
  Demux23/2 -> MATLAB Function6/2(u2)
  Demux23/1 -> MATLAB Function6/1(u1)
  Demux25/1 -> MATLAB Function11/1(u1)
  Demux25/2 -> MATLAB Function11/2(u2)
  SBI19/1 -> Demux25/1
  SBI18/1 -> Demux24/1
  Demux24/2 -> MATLAB Function5/2(u2)
  Demux24/1 -> MATLAB Function5/1(u1)
  Demux22/1 -> MATLAB Function12/1(u1)
  MATLAB Function9/1(y) -> Gain21/1
  MATLAB Function15/1(y) -> Gain18/1
  Demux27/1 -> MATLAB Function9/1(u1)
  Demux27/2 -> MATLAB Function9/2(u2)
  Demux28/1 -> MATLAB Function15/1(u1)
  SBI12/1 -> Demux26/1
  MATLAB Function7/1(y) -> Gain20/1
  Demux29/2 -> MATLAB Function16/2(u2)
  SBI14/1 -> Demux28/1
  MATLAB Function16/1(y) -> Gain19/1
  SBI13/1 -> Demux27/1
  Demux29/1 -> MATLAB Function16/1(u1)
  Demux26/2 -> MATLAB Function7/2(u2)
  Demux28/2 -> MATLAB Function15/2(u2)
  SBI15/1 -> Demux29/1
  Demux26/1 -> MATLAB Function7/1(u1)
  MATLAB Function17/1(y) -> Gain23/1
  Demux31/2 -> MATLAB Function17/2(u2)
  Demux31/1 -> MATLAB Function17/1(u1)
  MATLAB Function18/1(y) -> Gain22/1
  SBI17/1 -> Demux30/1
  Demux30/1 -> MATLAB Function18/1(u1)
  Demux30/2 -> MATLAB Function18/2(u2)
  SBI16/1 -> Demux31/1
  MATLAB Function20/1(y) -> Gain27/1
  MATLAB Function21/1(y) -> Gain24/1
  MATLAB Function19/1(y) -> Gain26/1
  MATLAB Function22/1(y) -> Gain25/1
  Demux32/1 -> MATLAB Function21/1(u1)
  Demux32/2 -> MATLAB Function21/2(u2)
  SBI20/1 -> Demux32/1
  SBI21/1 -> Demux33/1
  Demux33/2 -> MATLAB Function22/2(u2)
  Demux33/1 -> MATLAB Function22/1(u1)
  Demux35/1 -> MATLAB Function20/1(u1)
  Demux35/2 -> MATLAB Function20/2(u2)
  SBI23/1 -> Demux35/1
  SBI22/1 -> Demux34/1
  Demux34/2 -> MATLAB Function19/2(u2)
  Demux34/1 -> MATLAB Function19/1(u1)
  MATLAB Function25/1(y) -> Gain31/1
  MATLAB Function26/1(y) -> Gain28/1
  Demux37/1 -> MATLAB Function25/1(u1)
  Demux37/2 -> MATLAB Function25/2(u2)
  Demux38/1 -> MATLAB Function26/1(u1)
  SBI24/1 -> Demux36/1
  MATLAB Function24/1(y) -> Gain30/1
  Demux39/2 -> MATLAB Function27/2(u2)
  SBI26/1 -> Demux38/1
  MATLAB Function27/1(y) -> Gain29/1
  SBI25/1 -> Demux37/1
  Demux39/1 -> MATLAB Function27/1(u1)
  Demux36/2 -> MATLAB Function24/2(u2)
  Demux38/2 -> MATLAB Function26/2(u2)
  SBI27/1 -> Demux39/1
  Demux36/1 -> MATLAB Function24/1(u1)
  MATLAB Function28/1(y) -> Gain33/1
  Demux41/2 -> MATLAB Function28/2(u2)
  Demux41/1 -> MATLAB Function28/1(u1)
  MATLAB Function29/1(y) -> Gain32/1
  SBI29/1 -> Demux40/1
  Demux40/1 -> MATLAB Function29/1(u1)
  Demux40/2 -> MATLAB Function29/2(u2)
  SBI28/1 -> Demux41/1
  MATLAB Function31/1(y) -> Gain34/1
  Demux2/1 -> MATLAB Function31/1(u1)
  SBI9/1 -> Demux2/1
  Demux2/2 -> MATLAB Function31/2(u2)
  MATLAB Function30/1(y) -> Gain35/1
  SBI8/1 -> Demux4/1
  Demux4/1 -> MATLAB Function30/1(u1)
  Demux4/2 -> MATLAB Function30/2(u2)
  MATLAB Function33/1(y) -> Gain36/1
  Demux5/1 -> MATLAB Function33/1(u1)
  SBI11/1 -> Demux5/1
  Demux5/2 -> MATLAB Function33/2(u2)
  MATLAB Function32/1(y) -> Gain37/1
  SBI10/1 -> Demux7/1
  Demux7/2 -> MATLAB Function32/2(u2)
  Gain35/1 -> Probe/1
  Gain34/1 -> Probe5/1
  Gain36/1 -> Probe8/1
  Gain37/1 -> Probe6/1
  MATLAB Function35/1(y) -> Gain38/1
  Demux10/1 -> MATLAB Function35/1(u1)
  SBI37/1 -> Demux10/1
  Demux10/2 -> MATLAB Function35/2(u2)
  MATLAB Function34/1(y) -> Gain39/1
  SBI36/1 -> Demux11/1
  Demux11/1 -> MATLAB Function34/1(u1)
  Demux11/2 -> MATLAB Function34/2(u2)
  MATLAB Function37/1(y) -> Gain40/1
  Demux12/1 -> MATLAB Function37/1(u1)
  SBI35/1 -> Demux12/1
  MATLAB Function36/1(y) -> Gain41/1
  SBI34/1 -> Demux13/1
  Demux13/2 -> MATLAB Function36/2(u2)
  Gain39/1 -> Probe10/1
  Gain38/1 -> Probe11/1
  Gain40/1 -> Probe13/1
  Gain41/1 -> Probe12/1
  Demux7/1 -> MATLAB Function32/1(u1)
  Demux13/1 -> MATLAB Function36/1(u1)
  Demux12/2 -> MATLAB Function37/2(u2)
  MATLAB Function39/1(y) -> Gain42/1
  Demux16/1 -> MATLAB Function39/1(u1)
  SBI41/1 -> Demux16/1
  Demux16/2 -> MATLAB Function39/2(u2)
  MATLAB Function38/1(y) -> Gain43/1
  SBI40/1 -> Demux42/1
  Demux42/1 -> MATLAB Function38/1(u1)
  Demux42/2 -> MATLAB Function38/2(u2)
  MATLAB Function41/1(y) -> Gain44/1
  Demux43/1 -> MATLAB Function41/1(u1)
  SBI39/1 -> Demux43/1
  MATLAB Function40/1(y) -> Gain45/1
  SBI38/1 -> Demux44/1
  Demux44/2 -> MATLAB Function40/2(u2)
  Gain43/1 -> Probe14/1
  Gain42/1 -> Probe15/1
  Gain44/1 -> Probe21/1
  Gain45/1 -> Probe20/1
  Demux44/1 -> MATLAB Function40/1(u1)
  Demux43/2 -> MATLAB Function41/2(u2)

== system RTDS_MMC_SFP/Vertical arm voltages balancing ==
  note: The arm-level vertical energy balancing is done by acting on the circulating current of each leg in such a way that the total DC bus current is unchanged.
  theta : Inport
  acqdata : Inport  Port=2
  Kp_bal : Inport  Port=3
  Bus Selector1 : BusSelector  OutputSignals=A.Vsm.Vsm_up_avg,A.Vsm.Vsm_low_avg,B.Vsm.Vsm_up_avg,B.Vsm.Vsm_low_avg,C.Vsm.Vsm_up_avg,C.Vsm.Vsm_low_avg
  Constant : Constant  Value=[0 0 0]  OutDataTypeStr=single
  MATLAB Function : MATLAB Function  TreatAsAtomicUnit=on
  Mux : Mux  Inputs=2
  Mux1 : Mux  Inputs=3
  Scope : Scope
  Sum : Sum  Inputs=+-|
  Sum1 : Sum  Inputs=-+|
  Sum2 : Sum  Inputs=-+|
  Sum3 : Sum  Inputs=-+|
  vert_reg1 : simulink/Continuous/PID Controller  Controller=P  TimeDomain=Discrete-time  SampleTime=-1  IntegratorMethod=Forward Euler  FilterMethod=Forward Euler  Form=Parallel  UseFilter=on  ControllerParametersSource=external  P=0.2  I=0.5  D=0  N=100  InitialConditionSource=internal  InitialConditionForIntegrator=0  InitialConditionForFilter=0  ExternalReset=none  LimitOutput=off  UpperSaturationLimit=inf  LowerSaturationLimit=-inf  LinearizeAsGain=off  AntiWindupMode=none  Kb=1  TrackingMode=off  Kt=1  PParamMin=[]  PParamMax=[]  IParamMin=[]  IParamMax=[]  DParamMin=[]  DParamMax=[]  NParamMin=[]  NParamMax=[]  KbParamMin=[]  KbParamMax=[]  KtParamMin=[]  KtParamMax=[]  POutMin=[]  POutMax=[]  IOutMin=[]  IOutMax=[]  DOutMin=[]  DOutMax=[]  NOutMin=[]  NOutMax=[]  KbOutMin=[]  KbOutMax=[]  KtOutMin=[]  KtOutMax=[]  IntegratorOutMin=[]  IntegratorOutMax=[]  FilterOutMin=[]  FilterOutMax=[]  SumOutMin=[]  SumOutMax=[]  SumI1OutMin=[]  SumI1OutMax=[]  SumI2OutMin=[]  SumI2OutMax=[]  SumI3OutMin=[]  SumI3OutMax=[]  SumDOutMin=[]  SumDOutMax=[]  SaturationOutMin=[]  SaturationOutMax=[]  IntegratorContinuousStateAttributes=''  IntegratorStateMustResolveToSignalObject=off  IntegratorRTWStateStorageClass=Auto  FilterContinuousStateAttributes=''  FilterStateMustResolveToSignalObject=off  FilterRTWStateStorageClass=Auto  DifferentiatorICPrevScaledInput=0  DifferentiatorOutMin=[]  DifferentiatorOutMax=[]
  Ibal_abc : Outport
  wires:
  Sum1/1 -> Mux1/1  "Vert_unbal_A"
  Sum3/1 -> Mux1/3  "Vert_unbal_C"
  Sum2/1 -> Mux1/2  "Vert_unbal_B"
  theta/1 -> MATLAB Function/2(theta)
  vert_reg1/1 -> MATLAB Function/1(u)
  MATLAB Function/1(y) -> Ibal_abc/1
  Sum/1 -> vert_reg1/1
  Mux1/1 -> Mux/2, Sum/2
  Kp_bal/1 -> vert_reg1/2
  acqdata/1 -> Bus Selector1/1
  Bus Selector1/2 -> Sum1/2  "<Vsm_low_avg>"
  Bus Selector1/1 -> Sum1/1  "<Vsm_up_avg>"
  Bus Selector1/3 -> Sum2/1  "<Vsm_up_avg>"
  Bus Selector1/4 -> Sum2/2  "<Vsm_low_avg>"
  Bus Selector1/5 -> Sum3/1  "<Vsm_up_avg>"
  Bus Selector1/6 -> Sum3/2  "<Vsm_low_avg>"
  Constant/1 -> Mux/1, Sum/1
  Mux/1 -> Scope/1

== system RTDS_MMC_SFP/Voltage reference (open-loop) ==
  M_inv : Inport
  Vdc : Inport  Port=2
  Angle : BoomBox/PLLs/Angle  FREQ=fg  TSAMPLE_INT=CTRLPERIOD  UpLimit=pi  LowLimit=-pi  KBID=kb0702
  Constant : Constant  Value=0  OutDataTypeStr=single
  Mux : Mux  Inputs=3
  Probe : BoomBox/Probe  VARNAME=theta  EVALUATE=Literal  DATATYPE=single  CAN_ENABLED=off  CAN_ADDRESS=0  CAN_TX_FREQ=10  init_baudrate=0  CAN_BAUDRATE=1000000  can_endianness=Little-endian  ETH_ENABLED=off  ETH_PORT=2000  ETH_IP_LIST=IP address 0  eth_endianness=Little-endian  ETH_TX_FREQ=10  init_ip=0  KBID=kb0502  CAN_BIG_ENDIAN=0  ETH_BIG_ENDIAN=0  ETH_IP_SFCN=empty  CAN_MB_ID=0  ETH_MB_ID=1  RESIZE=0
  Product1 : Product
  Scope : Scope
  dq0 to abc1 : BoomBox/Transformations/dq0 to abc  KBID=kb0602
  Eabc_ref : Outport
  theta : Outport  Port=2
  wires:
  Vdc/1 -> Product1/2
  Product1/1 -> dq0 to abc1/1
  Mux/1 -> Product1/1
  Constant/1 -> Mux/2, Mux/3
  M_inv/1 -> Mux/1
  Angle/1 -> Probe/1, theta/1, dq0 to abc1/2
  dq0 to abc1/1 -> Scope/1, Eabc_ref/1
